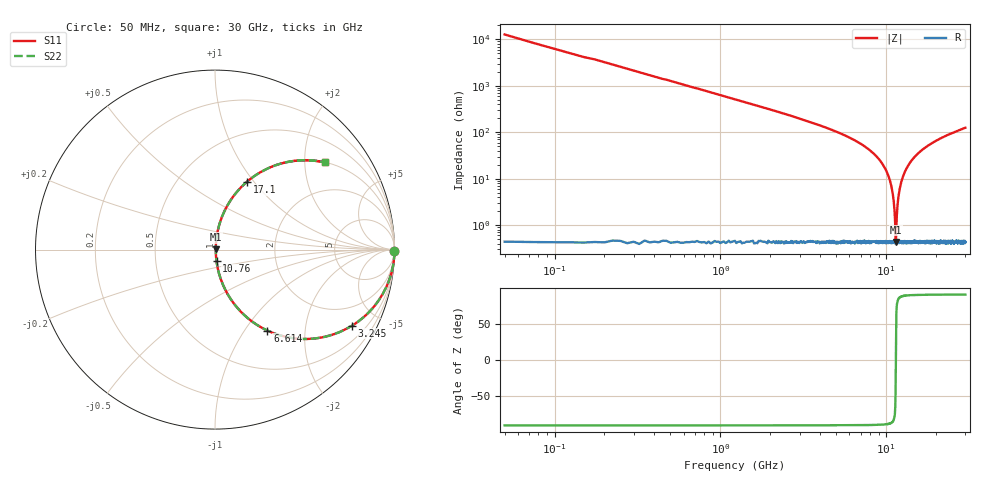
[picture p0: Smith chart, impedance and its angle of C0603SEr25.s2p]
!	AVX Thin Film Operation 	Date: April 2014
!	Description: Accu-P® Series, Thin Film  SMD RF Capacitor
!	Part Number: 06031JR25ZBSTR
# MHZ S MA R 50
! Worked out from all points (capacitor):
!   1201 points, 50 MHz to 30 GHz, reference 50 ohm
!   read as one part in series: C = 250 fF near 199.8 MHz
!   lowest |Z| = 433 mohm at 11.43 GHz (marker M1)
!   series resonance near 11.42 GHz, so ESL is about 780 pH
!   S11 on the Smith chart (normalised r, x): 50 MHz: open; 3.245 GHz: 1.01, -3.61; 6.614 GHz: 1.01, -1.28; 10.76 GHz: 1.01, -0.13; 17.1 GHz: 1.01, +0.92; 30 GHz: 1.01, +2.50
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50  1 -0.5  0.007854 89.5  0.007854 89.5  1 -0.5
374.458  0.998 -3.4  0.059 86.6  0.059 86.6  0.998 -3.4
873.625  0.991 -7.9  0.137 82.1  0.137 82.1  0.991 -7.9
1822.042  0.959 -16.4  0.282 73.6  0.282 73.6  0.959 -16.4
3244.667  0.874 -29.0  0.484 60.9  0.484 60.9  0.874 -29.0
5041.667  0.711 -44.4  0.7 45.3  0.7 45.3  0.711 -44.4
6614.042  0.537 -57.1  0.84 32.5  0.84 32.5  0.537 -57.1
8710.542  0.291 -72.3  0.953 16.9  0.953 16.9  0.291 -72.3
10058.29  0.14 -80.2  0.986 8.0  0.986 8.0  0.14 -80.2
10757.12  0.066 -82.5  0.994 3.8  0.994 3.8  0.066 -82.5
11056.62  0.036 -81.1  0.995 2.1  0.995 2.1  0.036 -81.1
11331.17  0.009622 -62.9  0.996 0.5  0.996 0.5  0.009622 -62.9
11431  0.00446 14.7  0.996 -0.1  0.996 -0.1  0.00446 14.7
11505.88  0.009428 62.3  0.996 -0.5  0.996 -0.5  0.009428 62.3
11855.29  0.042 81.7  0.995 -2.4  0.995 -2.4  0.042 81.7
12404.38  0.092 82.1  0.992 -5.3  0.992 -5.3  0.092 82.1
13452.62  0.18 78.3  0.979 -10.4  0.979 -10.4  0.18 78.3
15025  0.295 72.1  0.951 -17.1  0.951 -17.1  0.295 72.1
17096.54  0.418 64.7  0.904 -24.7  0.904 -24.7  0.418 64.7
20016.67  0.549 56.3  0.832 -33.3  0.832 -33.3  0.549 56.3
25033.29  0.694 45.8  0.717 -43.9  0.717 -43.9  0.694 45.8
30000  0.78 38.5  0.623 -51.3  0.623 -51.3  0.78 38.5
